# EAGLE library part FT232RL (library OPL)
USB UART IC Source: http://www.ftdichip.com/Documents/DataSheets/DS_FT232R_v104.pdf
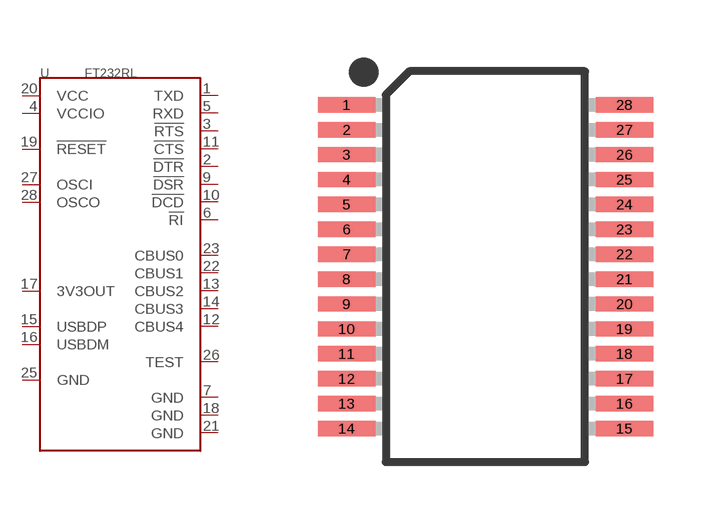
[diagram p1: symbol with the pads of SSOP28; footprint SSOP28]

Designator prefix U

## FT232RL-1720010P1  [SSOP28]
1  TXD  in
2  !DTR  in
3  !RTS  in
4  VCCIO  in
5  RXD  in
6  !RI  in
7  GND  in
9  !DSR  in
10  !DCD  in
11  !CTS  in
12  CBUS4  in
13  CBUS2  in
14  CBUS3  in
15  USBDP  in
16  USBDM  in
17  3V3OUT  in
18  GND  in
19  !RESET  in
20  VCC  in
21  GND  in
22  CBUS1  in
23  CBUS0  in
25  GND  in
26  TEST  in
27  OSCI  in
28  OSCO  in

## Footprint SSOP28 (pad centres in mm)
Shrink Small Outline Package SSOP-28 http://www.ftdichip.com/Documents/DataSheets/DS_FT232R_v104.pdf
smd 1.5 x 0.4: 1 -3.625,4.225; 2 -3.625,3.575; 3 -3.625,2.925; 4 -3.625,2.275; 5 -3.625,1.625; 6 -3.625,0.975; 7 -3.625,0.325; 8 -3.625,-0.325; 9 -3.625,-0.975; 10 -3.625,-1.625; 11 -3.625,-2.275; 12 -3.625,-2.925; 13 -3.625,-3.575; 14 -3.625,-4.225; 15 3.625,-4.225; 16 3.625,-3.575; 17 3.625,-2.925; 18 3.625,-2.275; 19 3.625,-1.625; 20 3.625,-0.975; 21 3.625,-0.325; 22 3.625,0.325; 23 3.625,0.975; 24 3.625,1.625; 25 3.625,2.275; 26 3.625,2.925; 27 3.625,3.575; 28 3.625,4.225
